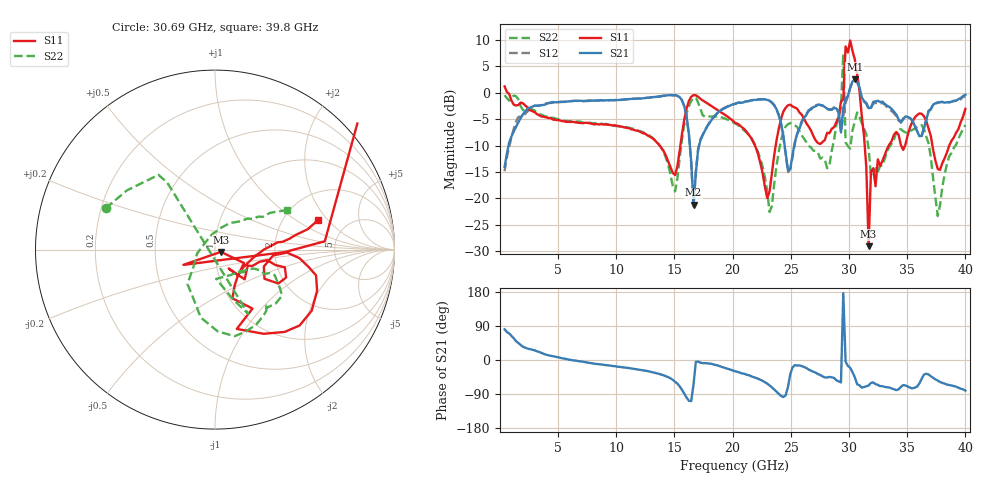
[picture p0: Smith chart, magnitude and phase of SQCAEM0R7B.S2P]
! Network Analyzer HP8722ES.07.66: Jul 25, 2000 Serial No. US39175408
! 26 Oct 2004  09:45:25
! Frequency  S11  S21  S12  S22
# HZ  S  DB R  50
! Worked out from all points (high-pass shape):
!   201 points, 400 MHz to 40 GHz, reference 50 ohm
!   highest |S21| = 2.57 dB at 30.5 GHz (marker M1); lowest = -21.2 dB at 16.64 GHz (marker M2)
!   |S21| within 3 dB of the highest: 14.64065 GHz to 14.67629 GHz (35.64 MHz wide, 0.243 % of centre); 29.92 GHz to 31.05 GHz (1.128 GHz wide, 3.7 % of centre)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
!   lowest |S11| = -29.1 dB at 31.68 GHz (marker M3), VSWR 1.07, Z = 53.4 - j1.35 ohm
!   |S11| at or under -10 dB: 13.73 GHz to 15.51 GHz (1.776 GHz wide, 12.1 % of centre); 21.91 GHz to 23.7 GHz (1.788 GHz wide, 7.84 % of centre); 31.35 GHz to 33.42 GHz (2.068 GHz wide, 6.38 % of centre)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
!   |S22| runs from -23.3 to 7.4 dB; largest |S21 - S12| = 0.17
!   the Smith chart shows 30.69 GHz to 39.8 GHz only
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4e8  1.20 -9.5  -14.02 81.0  -14.85 85.3  -0.44 -3.3
7.132e9  -5.75 -87.9  -1.55 -4.6  -1.59 -5.6  -5.66 -103.4
1.3666e10  -9.80 -96.9  -0.74 -36.5  -0.66 -36.8  -9.82 -154.5
1.5646e10  -7.75 -10.5  -1.42 -78.7  -1.42 -79.2  -8.77 16.0
1.6636e10  -0.42 -55.0  -21.22 -64.8  -21.54 -60.4  -0.97 -64.4
2.02e10  -5.69 -102.0  -2.15 -29.7  -2.06 -30.0  -5.79 -141.1
2.317e10  -18.69 -34.5  -1.48 -67.0  -1.55 -67.9  -22.58 94.6
2.4754e10  -2.36 -49.3  -14.72 -71.0  -15.02 -70.0  -5.94 -84.2
2.6932e10  -8.18 -88.9  -2.71 -31.0  -2.57 -31.8  -10.96 -173.9
2.8912e10  -5.53 -25.5  -2.96 -53.3  -3.01 -54.4  -6.10 97.5
2.9308e10  -1.66 -11.8  -7.53 -59.2  -7.37 -60.0  -2.74 39.2
2.9506e10  -1.23 -15.8  -2.90 176.6  -4.45 -172.2  7.41 18.7
2.9704e10  8.79 25.9  -1.22 -4.3  -1.93 1.9  -9.40 -35.3
2.9902e10  7.63 -59.9  -0.56 -15.6  -0.60 -16.4  -10.12 29.0
3.01e10  9.92 -76.9  0.95 -20.7  0.93 -20.8  -10.58 32.6
3.0496e10  6.32 -107.3  2.57 -45.6  2.46 -46.8  -5.47 0.5
3.0694e10  3.58 39.5  2.19 -63.8  2.06 -65.6  -3.73 159.3
3.1684e10  -29.06 -20.9  -2.91 -67.3  -3.08 -66.8  -10.57 -70.0
3.3466e10  -9.80 -13.1  -2.67 -72.7  -3.13 -74.0  -10.28 -26.3
3.6238e10  -3.97 -41.9  -8.15 -49.8  -8.21 -48.3  -6.11 -77.4
3.7624e10  -14.42 -47.1  -1.82 -54.4  -1.90 -55.8  -23.34 153.4
4e10  -3.04 15.1  -0.38 -80.8  -0.72 -80.5  -6.10 25.2
